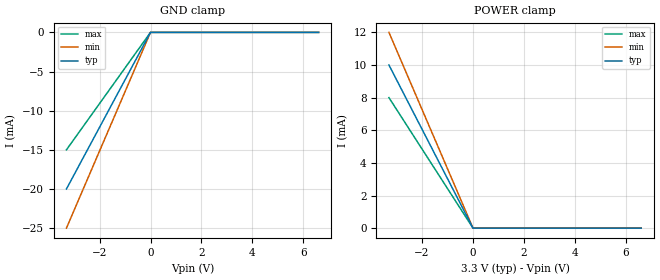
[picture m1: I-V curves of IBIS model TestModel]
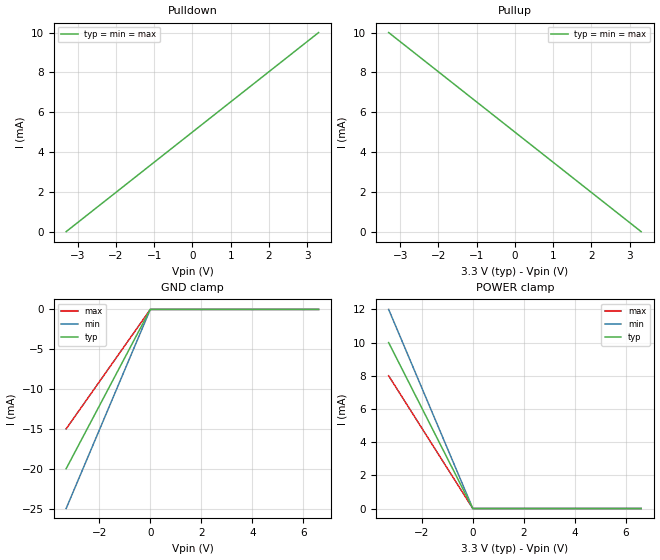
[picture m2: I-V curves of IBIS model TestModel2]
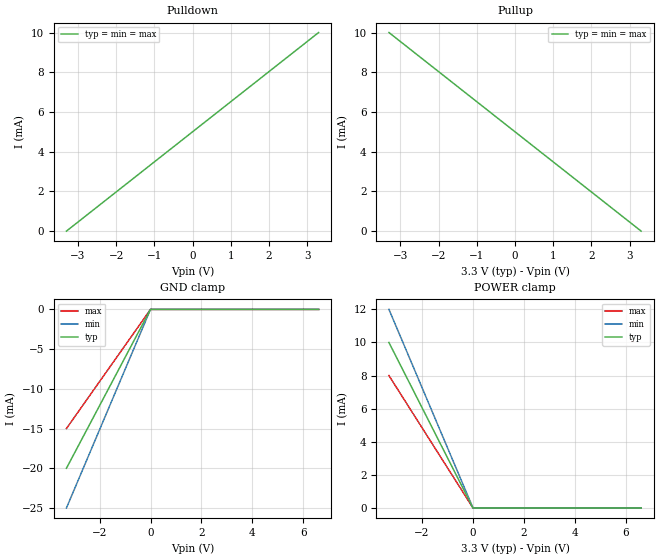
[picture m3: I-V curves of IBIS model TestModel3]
|DESCRIPTION OF BUG:
|The current parser allows models of type Input to include buffer delay fixture
|parameters (Vref, Rref, Cref) without generating a warning or error message.
|Additionally, no warning or error message is generated when Vmeas is present
|within a [Model Spec].  The presence of Vmeas outside of a [Model Spec]
|generates spurious warnings regarding the inability of the IV curves to cross
|through the Vmeas point using the selected Rref and Vref values.
|Some indication -- most appropriately, a warning -- should be made of the
|inconsistency between the buffer type and the use of buffer delay fixture
|data for such models.
|An example:
|  WARNING (line  xxx) - Output buffer delay fixture parameters (Vref, Cref,
|  Rref, Vmeas) are meaningless in buffers that can't be outputs (Model_type
|  Input, etc.)
|This warning should appear regardless of the presence or absence of [Model
|Spec] parameters.  No warnings should appear regarding inappropriate _values_
|of Rref, Vmeas and Vref within an Input model.
|This bug also applies to DOS32 IBISCHK3 v3.2.5.
[IBIS Ver]   3.2
[File Name]   bug48.ibs
[File Rev]   0.0
[Date]   02-November-2000
[Source]   File created from specification
[Disclaimer]
   (C) Copyright 2000 Intel Corp.
   All rights reserved
   This model is for demonstration purposes only,
[Component]   GENERIC_IBIS
[Manufacturer]   Intel Corp.
[Package]
|   typ   min   max
R_pkg   6.0mO   5.0mO   7.0mO
L_pkg   5.0nH   2.0nH   8.0nH
C_pkg   1.0pF   0.5pF   1.5pF
[Pin]   signal_name   model_name   R_pin   L_pin   C_pin
   1   TestSignal1   TestModel
   2   TestSignal2   TestModel2
   3   TestSignal3   TestModel3
   4   TestSignal4   TestModel4
   5   TestSignal5   TestModel5
[Model]   TestModel5
Model_type   Terminator
C_comp   5.00pF   4.00pF   6.00pF
| ... all of these should generate warnings for a Terminator type
Cref = 10.0pF
Vref = 0.0
Rref = 25
[Model Spec]
| ... all of these should generate warnings for a Terminator type
Vmeas   1.3   1.2   1.5
Vinl   1   NA   NA
Vinh   1   NA   NA
Vinl+   1   NA   NA
Vinl-   1   NA   NA
Vinh+   1   NA   NA
Vinh-   1   NA   NA
D_overshoot_high   .2   NA   NA
D_overshoot_low   -0.2   NA   NA
S_overshoot_low   -0.1   NA   NA
S_overshoot_high   .1   NA   NA
D_overshoot_time   1n   NA   NA
Pulse_high   3   NA   NA
Pulse_low   0.5   NA   NA
Pulse_time   1n   NA   NA
[Temperature Range]   27.00   100.00   0.00
[Voltage Range]   3.30V   3.00V   3.60V
| Models and submodels in the file (5): TestModel (Input), TestModel2 (Output), TestModel3 (Output), TestModel4 (I/O), TestModel5 (Terminator)
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[Model]   TestModel
Model_type   Input
Vinl = 800mV
Vinh = 2.0V
| ... These should generate warnings for an input model type
Cref = 10.0pF
Vref = 0.0
Rref = 25
Vmeas = 1.4
C_comp   5.00pF   4.00pF   6.00pF
[Model Spec]
| ... this is not OK for an input model type
Vmeas   1.3   1.2   1.5
| ... these are  OK for an input model type
Vinl   1   NA   NA
Vinh   1   NA   NA
Vinl+   1   NA   NA
Vinl-   1   NA   NA
Vinh+   1   NA   NA
Vinh-   1   NA   NA
D_overshoot_high   .2   NA   NA
D_overshoot_low   -0.2   NA   NA
S_overshoot_low   -0.1   NA   NA
S_overshoot_high   .1   NA   NA
D_overshoot_time   1n   NA   NA
Pulse_high   3   NA   NA
Pulse_low   0.5   NA   NA
Pulse_time   1n   NA   NA
[Temperature Range]   27.00   100.00   0.00
[Voltage Range]   3.30V   3.00V   3.60V
[GND Clamp]
| voltage   I(typ)   I(min)   I(max)
-3.3V     -20mA      -25mA      -15mA
0V        0A         -5nA       -5nA
3.3V      0A         0A         0A
6.6V      0A         0A         0A
[Power Clamp]
| voltage   I(typ)   I(min)   I(max)
-3.3V     10mA       12mA       8mA
0V        0A         300nA      300nA
3.3V      0A         0A         0A
6.6V      0A         0A         0A
[Model]   TestModel2
Model_type   Output
Polarity   Non-Inverting
| ... these are OK for an Output model type
Cref = 10.0pF
Vref = 0.0
Rref = 25
| ... this Vmeas should be used when checking the drive of the model
Vmeas = 1.4
C_comp   5.00pF   4.00pF   6.00pF
[Temperature Range]   27.00   100.00   0.00
[Voltage Range]   3.30V   3.00V   3.60V
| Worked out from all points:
|   slope of the pulldown table from 0 to 0.495 V, typ, clamps not added: 660 ohm
|   slope of the pullup table from 0 to 0.495 V, typ, clamps not added: 660 ohm
[GND Clamp]
| voltage   I(typ)   I(min)   I(max)
-3.3V     -20mA      -25mA      -15mA
0V        0A         -5nA       -5nA
3.3V      0A         0A         0A
6.6V      0A         0A         0A
[Power Clamp]
| voltage   I(typ)   I(min)   I(max)
-3.3V     10mA       12mA       8mA
0V        0A         300nA      300nA
3.3V      0A         0A         0A
6.6V      0A         0A         0A
[Pullup]
-3.3V     10mA       10mA       10mA
3.3V      0A         0A         0A
[Pulldown]
-3.3V     0A         0A         0A
3.3V      10mA       10mA       10mA
[Ramp]
dV/dt_r   1.5/.6n NA NA
dV/dt_f   1.5/.6n NA NA
[Model]   TestModel3
Model_type   Output
Polarity   Non-Inverting
| ... these should generate a warning for Output model types
Vinl = 800mV
Vinh = 2.0V
| ... These are Ok for an Output model type
Cref = 10.0pF
Vref = 0.0
Rref = 25
| ... The model spec Vmeas will be used for checking the drive of the curves
| ... This should be ignored
Vmeas = 1.4
C_comp   5.00pF   4.00pF   6.00pF
[Model Spec]
| ... this is OK for an output model type
| ... and should be used to check the output drive
Vmeas   1.3   1.2   1.5
| ... these are not OK for an output model type
Vinl   1   NA   NA
Vinh   1   NA   NA
Vinl+   1   NA   NA
Vinl-   1   NA   NA
Vinh+   1   NA   NA
Vinh-   1   NA   NA
D_overshoot_high   .2   NA   NA
D_overshoot_low   -0.2   NA   NA
S_overshoot_low   -0.1   NA   NA
S_overshoot_high   .1   NA   NA
D_overshoot_time   1n   NA   NA
Pulse_high   3   NA   NA
Pulse_low   0.5   NA   NA
Pulse_time   1n   NA   NA
[Temperature Range]   27.00   100.00   0.00
[Voltage Range]   3.30V   3.00V   3.60V
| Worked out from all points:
|   slope of the pulldown table from 0 to 0.495 V, typ, clamps not added: 660 ohm
|   slope of the pullup table from 0 to 0.495 V, typ, clamps not added: 660 ohm
[GND Clamp]
| voltage   I(typ)   I(min)   I(max)
-3.3V     -20mA      -25mA      -15mA
0V        0A         -5nA       -5nA
3.3V      0A         0A         0A
6.6V      0A         0A         0A
[Power Clamp]
| voltage   I(typ)   I(min)   I(max)
-3.3V     10mA       12mA       8mA
0V        0A         300nA      300nA
3.3V      0A         0A         0A
6.6V      0A         0A         0A
[Pullup]
-3.3V     10mA       10mA       10mA
3.3V      0A         0A         0A
[Pulldown]
-3.3V     0A         0A         0A
3.3V      10mA       10mA       10mA
[Ramp]
dV/dt_r   1.5/.6n NA NA
dV/dt_f   1.5/.6n NA NA
